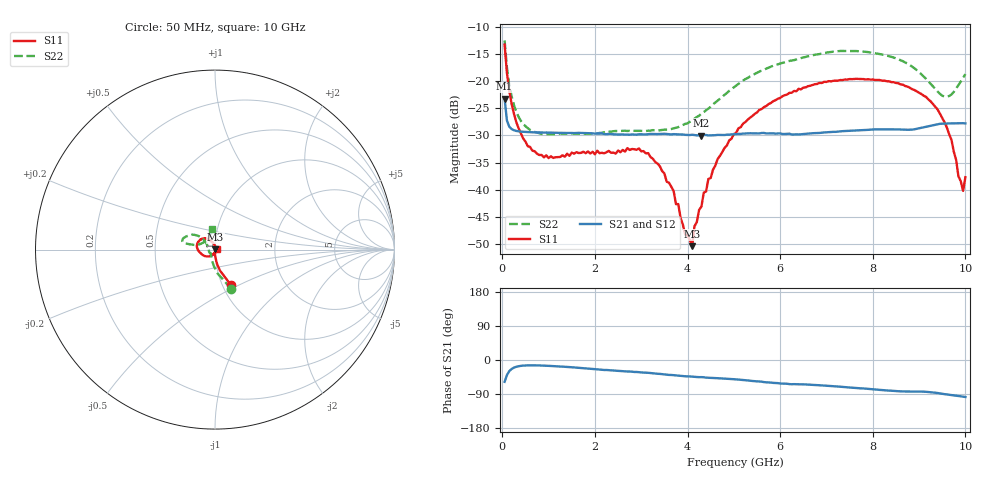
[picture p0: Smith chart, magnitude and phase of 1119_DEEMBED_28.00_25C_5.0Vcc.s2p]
!Hittite Microwave Corp.
!Digital Attenuator/PhaseShifter Rev 1.4.0
!Filename: C:\DATA\DATA\1119_DEEMBED_28.00_25C_5.0Vcc.s2p
!VNA ID: Agilent Technologies,N5224A,MY51441122,A.10.45.03
!Device type:
!2 Port Calibration.
!Temp(C): 25
!Lot Number:
!Serial Number:
!Operator:
!Misc:
!Attenuator:  28.000
# GHZ S DB R 50.0
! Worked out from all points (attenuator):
!   200 points, 50 MHz to 10 GHz, reference 50 ohm
!   highest |S21| = -23.24 dB at 50 MHz (marker M1); lowest = -30.0 dB at 4.3 GHz (marker M2)
!   lowest |S11| = -50.3 dB at 4.1 GHz (marker M3), VSWR 1.01, Z = 50.3 + j0.156 ohm
!   |S11| at or under -10 dB: start of sweep to end of sweep
!   |S22| runs from -29.8 to -12.6 dB; largest |S21 - S12| = 0.00015
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0.05  -13.30 -65.8  -23.24 -57.6  -23.25 -57.6  -12.55 -67.5
0.1  -18.52 -76.9  -27.26 -39.9  -27.24 -39.9  -17.51 -84.0
0.2  -24.14 -84.0  -28.82 -23.8  -28.83 -23.7  -22.78 -100.6
0.55  -31.97 -91.0  -29.39 -14.2  -29.37 -14.2  -28.66 -126.4
1  -34.16 -97.0  -29.48 -15.4  -29.48 -15.5  -29.74 -137.3
1.75  -32.99 -105.3  -29.56 -21.7  -29.56 -21.7  -29.67 -140.8
2.95  -32.38 -93.4  -29.78 -32.0  -29.79 -32.1  -29.14 -160.2
3.4  -35.62 -90.4  -29.73 -36.6  -29.74 -36.7  -29.04 -173.7
3.7  -40.19 -77.7  -29.76 -40.1  -29.76 -40.2  -28.69 175.1
3.95  -48.21 -40.8  -29.89 -43.0  -29.90 -43.1  -27.87 164.0
4.1  -50.34 30.8  -29.87 -44.0  -29.89 -44.1  -27.18 158.1
4.15  -46.68 26.6  -29.93 -44.8  -29.93 -44.9  -26.93 155.8
4.3  -43.08 68.5  -30.01 -45.2  -30.02 -45.3  -25.99 150.4
4.65  -34.32 88.7  -29.90 -48.0  -29.91 -48.1  -23.63 141.8
5.05  -29.52 102.5  -29.75 -51.1  -29.77 -51.1  -20.84 138.6
5.75  -24.23 120.3  -29.63 -59.1  -29.64 -59.2  -17.55 143.1
6.7  -20.72 139.2  -29.59 -65.8  -29.60 -65.7  -15.26 153.8
8.35  -20.05 175.8  -28.89 -80.6  -28.89 -80.6  -15.43 168.1
9.400001  -25.25 -135.8  -27.95 -87.1  -27.95 -87.1  -21.92 153.7
9.7  -30.83 -107.4  -27.78 -92.5  -27.79 -92.6  -22.47 119.7
9.95  -40.18 -9.0  -27.75 -96.8  -27.76 -96.8  -19.43 100.0
10  -37.67 11.5  -27.79 -97.7  -27.79 -97.7  -18.73 98.2
